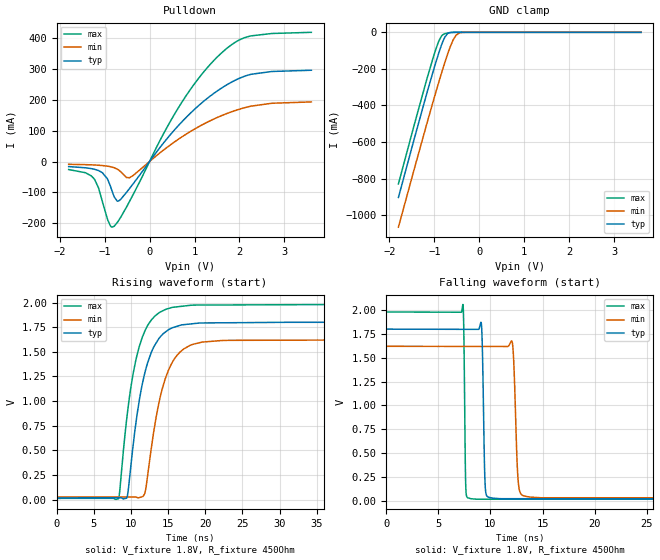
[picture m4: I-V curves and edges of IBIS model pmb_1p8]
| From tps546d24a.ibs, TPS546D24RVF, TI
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|   pmb_1p8 Model
[Model]   pmb_1p8
Model_type   I/O_open_drain
Polarity   Inverting
Enable   Active-High
Vinl = 0.8
Vinh = 1.35
Vmeas = 0.9
Vref = 1.8
Cref = 2pF
Rref = 450
|   typ   min   max
C_comp   3.562pF   3.480pF   3.661pF
|C_comp_pull_down   4.165pF   4.033pF   4.567pF
|  Where Nom  PVT is Nominal Process, 1.8V,  25C
|   Fast PVT is Strong Process,  1.89V, -40C
|   Slow PVT is Weak Process,   1.62V, 150C
[Voltage Range]   1.8   1.62   1.98
|Junction Temperature
[Temperature Range]   25   150   -40
[Pullup Reference]   1.8   1.62   1.98
[Pulldown Reference]   0   0   0
[Power Clamp Reference]   1.8   1.62   1.98
[GND Clamp Reference]   0   0   0
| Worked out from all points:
|   slope of the pulldown table from 0 to 0.27 V, typ, clamps not added: 5.14 ohm
|   GND clamp passes 1 mA (typ) near -0.62 V on its own axis
|   falling waveform, V_fixture 1.8V, R_fixture 450Ohm: 20-80 % time 172ps typ, 289ps min, 118ps max; typ from 1.8 V to 0.019 V
|   rising waveform, V_fixture 1.8V, R_fixture 450Ohm: 20-80 % time 2.46ns typ, 2.56ns min, 2.39ns max; typ from 0.019 V to 1.8 V
[Pulldown]
|   Voltage   I(typ)   I(min)   I(max)
-1.8V     -16.54mA   -9.07mA    -26.12mA
-1.233V   -24.96mA   -11.31mA   -56.21mA
-1.136V   -29.43mA   -12.14mA   -85.72mA
-925.2mV  -60.25mA   -15.41mA   -191.6mA
-790.2mV  -113.5mA   -20.17mA   -210.4mA
-693mV    -128.4mA   -27.2mA    -192.6mA
-444.6mV  -87.39mA   -52.66mA   -129.2mA
613.8mV   112.2mA    69.51mA    167.9mA
1.067V    178.3mA    110.8mA    265.5mA
1.51V     229.4mA    143.1mA    339.7mA
2.207V    281mA      178mA      405.8mA
3.6V      296.1mA    193.4mA    419.2mA
[GND Clamp]
|   Voltage   I(typ)   I(min)   I(max)
-1.8V     -903.3mA   -1.066A    -829.2mA
-1.19V    -352.7mA   -519.2mA   -275.5mA
-1.017V   -204.7mA   -369.5mA   -130.3mA
-909mV    -118.2mA   -278.6mA   -52.68mA
-828mV    -60.58mA   -212.5mA   -16.63mA
-763.2mV  -24.67mA   -161.7mA   -7.231mA
-703.8mV  -6.599mA   -117.7mA   -3.401mA
-590.4mV  -325.4uA   -45.68mA   -375.9uA
-520.2mV  -52.37uA   -16.36mA   -59.09uA
-444.6mV  -6.312uA   -3.129mA   -5.317uA
-331.2mV  -146.2nA   -156.2uA   -36.62nA
3.6V      0A         0A         0A
[POWER Clamp]
|   Voltage   I(typ)   I(min)   I(max)
-1.8V     0A         0A         0A
0V        0A         0A         0A
3.6V      0A         0A         0A
[Ramp]
R_load = 450
|   typ   min   max
dV/dt_r   1.06835/2.449e-09   0.955095/2.55732e-09   1.17945/2.37954e-09
dV/dt_f   1.06835/1.72466e-10   0.955095/2.88482e-10   1.17945/1.18046e-10
[Falling Waveform]
V_fixture = 1.8V
V_fixture_min = 1.62V
V_fixture_max = 1.98V
R_fixture = 450Ohm
C_fixture = 0F
|   Time   V(typ)   V(min)   V(max)
0s        1.8V       1.62V      1.98V
7.357ns   1.798V     1.619V     2.058V
7.656ns   1.798V     1.619V     91.73mV
8.662ns   1.798V     1.618V     15.58mV
9.15ns    1.832V     1.618V     15.58mV
9.549ns   89.45mV    1.618V     15.58mV
10.98ns   20.89mV    1.618V     15.57mV
12.82ns   20.89mV    95.28mV    15.57mV
14.83ns   20.88mV    30.72mV    15.56mV
500ns     19.42mV    28.17mV    14.25mV
[Rising Waveform]
V_fixture = 1.8V
V_fixture_min = 1.62V
V_fixture_max = 1.98V
R_fixture = 450Ohm
C_fixture = 0F
|   Time   V(typ)   V(min)   V(max)
0s        19.42mV    28.17mV    14.25mV
8.348ns   20.1mV     28.17mV    11.65mV
9.526ns   36.54mV    28.17mV    875.5mV
10.66ns   767.8mV    27.82mV    1.413V
11.64ns   1.21V      34.01mV    1.668V
12.01ns   1.325V     111.9mV    1.732V
12.89ns   1.52V      597.4mV    1.835V
14.59ns   1.697V     1.219V     1.927V
18.13ns   1.784V     1.57V      1.973V
500ns     1.8V       1.62V      1.98V
